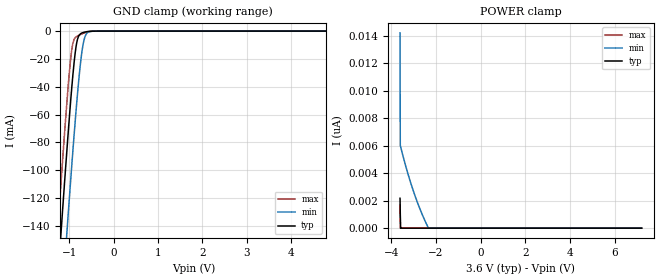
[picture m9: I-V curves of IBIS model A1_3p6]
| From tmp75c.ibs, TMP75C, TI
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|   Model
[Model]   A1_3p6
Model_type   Input
Vinl = 0.9
Vinh = 2.1
|   typ   min   max
C_comp   0.319pF   0.314pF   0.326pF
[Voltage Range]   3.6   3.59   3.61
[Temperature Range]   25   125   -40
[Power Clamp Reference]   3.6   3.59   3.61
[GND Clamp Reference]   0   0   0
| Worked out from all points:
|   GND clamp passes 1 mA (typ) near -0.68 V on its own axis
[GND Clamp]
|   Voltage   I(typ)   I(min)   I(max)
-3.6V     -1.323A    -1.379A    -1.29A
-1.278V   -187mA     -247.1mA   -151mA
-1.192V   -147mA     -207mA     -111mA
-1.181V   -142mA     -202mA     -106.1mA
-1.094V   -103mA     -162.6mA   -67.73mA
-1.03V    -74.89mA   -133.6mA   -40.99mA
-943.2mV  -40.15mA   -96.06mA   -13.07mA
-835.2mV  -8.827mA   -52.55mA   -3.897mA
-716.4mV  -1.383mA   -15.13mA   -2.039mA
-619.2mV  -502.6uA   -2.225mA   -893uA
-478.8mV  -65.18uA   -114.9uA   -103.9uA
7.2V      0A         0A         0A
[POWER Clamp]
|   Voltage   I(typ)   I(min)   I(max)
-3.6V     2.172nA    14.2nA     1.677nA
-3.589V   1.086nA    6.031nA    838.7pA
-3.578V   0A         5.959nA    0A
-3.298V   0A         4.241nA    0A
-2.995V   0A         2.663nA    0A
-2.693V   0A         1.329nA    0A
-2.336V   0A         25.09pA    0A
7.2V      0A         0A         0A
